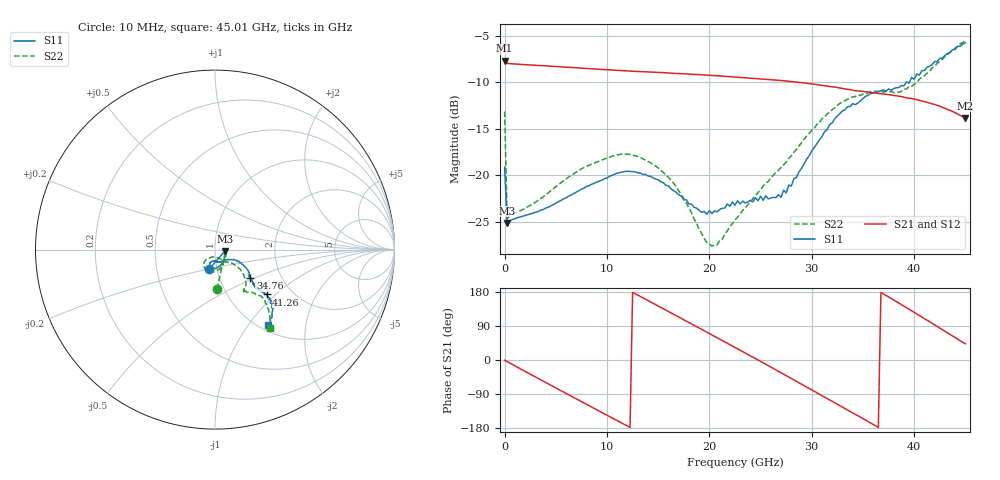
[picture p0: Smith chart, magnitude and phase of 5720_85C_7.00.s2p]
! Device:  ADRF5720
! Description: 0.5dB LSB GaAs MMIC 6-bit Digital Attenuator
! Frequency:  0.000009 -  40 GHz
! Ports:
!	RF1	= Port 1
!	RF2	= Port 2
! Vdd:  3.3 Volt
! Vss:  -3.3 Volt
! Control:  0/3.3 Volt
! State:  7.00 dB attenuation
! Data:  The device was measured using G-S-G Probes on a matrix board.
!  Data was collected using an calibrated 4 port network analyzer.
!  The reference plane for this measurement is at the launchers.
! Note:  Analog Devices supplies this data as a sample of measured data
!  for this product.  Your particular data for this product may vary.
!  Data was taken at 85 degrees C.
!  Analog Devices reserves the right to change this data at anytime.
# GHZ S DB R 45.0
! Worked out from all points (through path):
!   181 points, 10 MHz to 45.01 GHz, reference 45 ohm
!   highest |S21| = -7.66 dB at 10 MHz (marker M1); lowest = -13.8 dB at 45.01 GHz (marker M2)
!   group delay of S21, straight-line fit = 41.4 ps
!   lowest |S11| = -25.1 dB at 260 MHz (marker M3), VSWR 1.12, Z = 50.2 - j0.876 ohm
!   |S11| at or under -10 dB: start of sweep to 39.23 GHz; 39.36 GHz to 39.54629 GHz (186.3 MHz wide, 0.472 % of centre)
!   |S22| runs from -27.6 to -5.5 dB; largest |S21 - S12| = 0.0021
!   S11 on the Smith chart (normalised r, x): 10 MHz: 0.92, -0.20; 34.76 GHz: 1.40, -0.47; 41.26 GHz: 1.50, -0.88; 45.01 GHz: 1.09, -1.26
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0.01  -19.10 -106.1  -7.66 -0.7  -7.65 -0.7  -13.13 -87.0
0.26  -25.10 -9.0  -7.96 -4.0  -7.95 -4.0  -24.63 -8.8
2.26  -24.22 -18.0  -8.12 -33.8  -8.10 -33.7  -23.38 -23.8
4.26  -23.43 -37.9  -8.25 -62.9  -8.23 -62.8  -21.89 -48.2
6.01  -22.41 -50.0  -8.37 -88.2  -8.35 -88.1  -20.38 -63.5
7.76  -21.37 -60.9  -8.49 -113.4  -8.47 -113.3  -19.16 -76.2
9.76  -20.35 -75.1  -8.63 -142.2  -8.61 -142.0  -18.23 -91.2
11.51  -19.62 -86.8  -8.74 -167.2  -8.73 -167.1  -17.70 -102.8
13.26  -19.74 -97.9  -8.84 167.7  -8.83 167.9  -18.07 -114.2
15.26  -20.68 -107.6  -8.95 138.9  -8.93 139.0  -19.44 -125.8
17.76  -22.62 -108.2  -9.10 102.7  -9.08 102.9  -22.96 -130.6
20.26  -24.10 -91.0  -9.26 66.2  -9.24 66.3  -27.60 -98.5
22.76  -22.73 -75.4  -9.45 29.5  -9.43 29.7  -24.48 -60.6
24.76  -22.73 -68.3  -9.61 -0.0  -9.59 0.2  -21.83 -51.0
27.01  -22.34 -49.0  -9.80 -33.6  -9.78 -33.3  -19.14 -40.7
30.26  -16.98 -28.0  -10.22 -82.7  -10.20 -82.4  -14.92 -38.3
33.01  -13.06 -32.6  -10.66 -124.6  -10.64 -124.3  -12.08 -46.3
34.76  -11.98 -38.7  -10.93 -150.9  -10.92 -150.6  -11.41 -52.7
37.76  -10.84 -41.9  -11.37 162.4  -11.35 162.7  -10.99 -54.9
41.26  -8.38 -40.9  -12.14 105.1  -12.12 105.4  -9.04 -46.1
43.01  -7.11 -43.5  -12.78 75.9  -12.75 76.3  -7.25 -48.0
45.01  -5.75 -54.8  -13.83 42.6  -13.80 43.0  -5.50 -55.0
